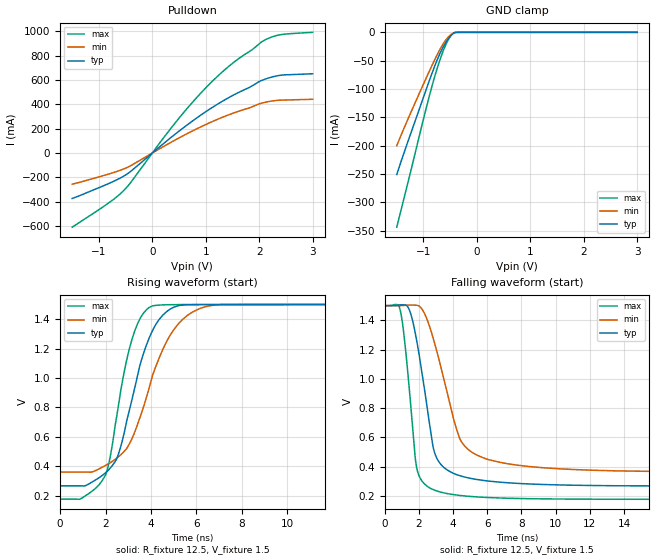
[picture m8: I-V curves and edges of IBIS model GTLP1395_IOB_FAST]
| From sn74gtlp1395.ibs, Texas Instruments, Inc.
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[Model]   GTLP1395_IOB_FAST
Model_type  I/O_open_drain
Vinl = 0.95
Vinh = 1.05
Enable   Active-Low
Vref =   1.5
Rref =   12.5
Cref =   30p
Vmeas =   1.0
| variable   typ   min   max
C_comp   7.53pF   6.02pF   8.49pF
| C_pulldown   9.41pF   5.85pF   15.57pF
| C_tri-state   7.53pF   6.02pF   8.49pF
[Temperature Range]   40   100   -40
| Ambient temperature   25   85   -40
[Voltage range]   1.5   1.5   1.5
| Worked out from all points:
|   slope of the pulldown table from 0 to 0.225 V, typ, clamps not added: 2.7 ohm
|   GND clamp passes 1 mA (typ) near -0.42 V on its own axis
|   rising waveform, R_fixture 12.5, V_fixture 1.5: 20-80 % time 1.24ns typ, 1.61ns min, 940ps max; typ from 0.267 V to 1.5 V
|   falling waveform, R_fixture 12.5, V_fixture 1.5: 20-80 % time 994ps typ, 1.56ns min, 618ps max; typ from 1.5 V to 0.267 V
[GND Clamp]
| GTLP1395_IOB_FAST
|   Voltage   I(typ)   I(min)   I(max)
-1.5V     -251mA     -200.2mA   -343.9mA
-1.325V   -202mA     -160.6mA   -278.1mA
-980mV    -109.1mA   -87.16mA   -145.5mA
-880mV    -82.51mA   -66.47mA   -108.8mA
-800mV    -62.2mA    -50.39mA   -81.3mA
-695mV    -38.08mA   -30.87mA   -49.54mA
-610mV    -22.36mA   -17.3mA    -27.87mA
-525mV    -10.04mA   -7.253mA   -11.29mA
-450mV    -2.617mA   -1.767mA   -2.187mA
-410mV    -522.4uA   -344.4uA   -180.8uA
-355mV    -26.7uA    -53.58uA   -21.94uA
3V        1.146nA    5.211nA    8.435nA
[Pulldown]
| GTLP1395_IOB_FAST
|   Voltage   I(typ)   I(min)   I(max)
-1.5V     -373.9mA   -256.1mA   -609.8mA
-835mV    -254.7mA   -175.4mA   -415.9mA
-530mV    -188.7mA   -129.9mA   -306.1mA
-405mV    -151.2mA   -104.3mA   -242.4mA
280mV     103.2mA    71.14mA    164.8mA
640mV     227.1mA    156.7mA    360.7mA
1.065V    358.5mA    247.4mA    565mA
1.465V    464.1mA    320.2mA    725.2mA
2.04V     595.6mA    409.6mA    912.6mA
2.205V    621.2mA    425.6mA    949.4mA
2.435V    641.6mA    435.6mA    976.1mA
3V        652.1mA    442.2mA    993.1mA
[Ramp]
| GTLP1395_IOB_FAST
| variable   typ   min   max
dV/dt_r   0.74/1.32E-09   0.68/1.67E-09   0.79/9.88E-10
dV/dt_f   0.74/1.01E-09   0.69/1.57E-09   0.80/6.26E-10
R_load = 12.5
[Rising Waveform]
| GTLP1395_IOB_FAST
R_fixture =   12.5
C_fixture =   0
L_fixture =   0
V_fixture =   1.5
V_fixture_min = 1.5
V_fixture_max = 1.5
|   Time   V(typ)   V(min)   V(max)
0s        267.4mV    361.4mV    177.7mV
910ps     267.2mV    361.3mV    179.7mV
2.02ns    359.3mV    408.1mV    347.6mV
2.535ns   469.6mV    460.5mV    781.4mV
3.095ns   810.2mV    566.4mV    1.225V
3.54ns    1.1V       742.4mV    1.409V
4.045ns   1.315V     1.004V     1.489V
5.165ns   1.49V      1.36V      1.499V
6.66ns    1.5V       1.493V     1.5V
25ns      1.5V       1.5V       1.5V
[Falling Waveform]
| GTLP1395_IOB_FAST
R_fixture =   12.5
C_fixture =   0
L_fixture =   0
V_fixture =   1.5
V_fixture_min = 1.5
V_fixture_max = 1.5
|   Time   V(typ)   V(min)   V(max)
0s        1.5V       1.5V       1.5V
885ps     1.505V     1.5V       1.478V
1.13ns    1.505V     1.501V     1.294V
1.48ns    1.459V     1.504V     873.2mV
1.9ns     1.241V     1.502V     377.4mV
2.735ns   604.3mV    1.317V     249.4mV
3.2ns     428.4mV    1.12V      229.3mV
4.37ns    340.1mV    597.7mV    204.6mV
5.77ns    306.7mV    461mV      191.7mV
25ns      267.5mV    362.3mV    177.7mV
